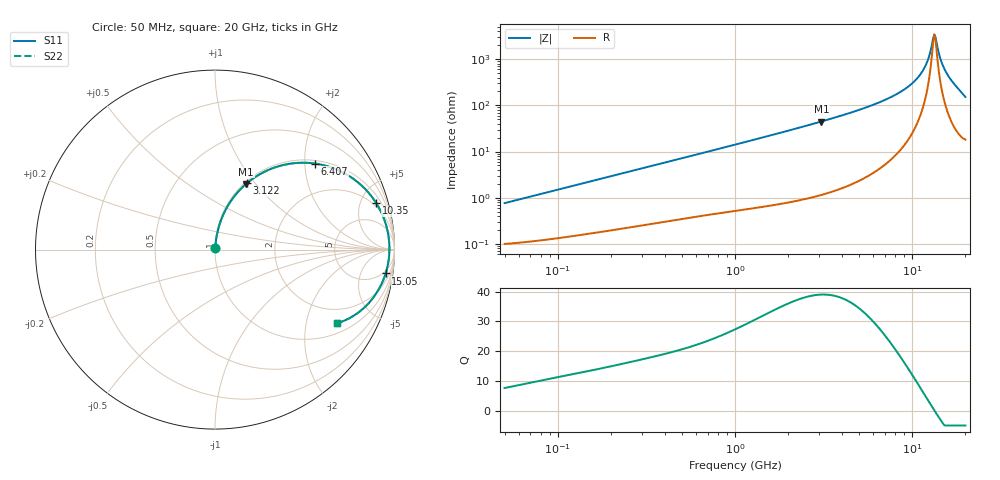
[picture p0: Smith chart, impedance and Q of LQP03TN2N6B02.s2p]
!Murata Part Number: LQP03TN2N6B02
!These Parameters are Measured in Series Mode Connection
!  o--[Z]--o
!Port1  Port2
!  o-------o
!Freq. Start=50[MHz] Stop=20[GHz], 401[Steps]
# Hz S RI R 50
!Freq.(Hz) S11(Real) S11(Imag) S21(Real) S21(Imag) S12(Real) S12(Imag) S22(Real) S22(Imag)
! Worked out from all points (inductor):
!   401 points, 50 MHz to 20 GHz, reference 50 ohm
!   read as one part in series: L = 2.4 nH near 51.52 MHz
!   highest Q = 39 at 3.075 GHz (marker M1), where L = 2.32 nH
!   self-resonance near 13.35 GHz
!   S11 on the Smith chart (normalised r, x): 50 MHz: 1.00, +0.02; 3.122 GHz: 1.02, +0.91; 6.407 GHz: 1.08, +2.26; 10.35 GHz: 1.63, +6.73; 15.05 GHz: 4, -13; 20 GHz: 1.36, -3.02
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5e7  0.00105 0.00755  0.9989 -0.00755  0.9989 -0.00755  0.00105 0.00755
1.364002e8  0.00198 0.0201  0.998 -0.0201  0.998 -0.0201  0.00198 0.0201
3.721004e8  0.0057 0.053  0.9943 -0.053  0.9943 -0.053  0.0057 0.053
1e9  0.0243 0.1367  0.9757 -0.1367  0.9757 -0.1367  0.0243 0.1367
2.728004e9  0.1401 0.3344  0.8599 -0.3344  0.8599 -0.3344  0.1401 0.3344
3.075291e9  0.1732 0.3658  0.8268 -0.3658  0.8268 -0.3658  0.1732 0.3658
3.121702e9  0.1778 0.3697  0.8222 -0.3697  0.8222 -0.3697  0.1778 0.3697
4.472136e9  0.3271 0.4556  0.6729 -0.4556  0.6729 -0.4556  0.3271 0.4556
6.406762e9  0.5583 0.4792  0.4417 -0.4792  0.4417 -0.4792  0.5583 0.4792
7.442007e9  0.672 0.4485  0.328 -0.4485  0.328 -0.4485  0.672 0.4485
8.907419e9  0.8058 0.3667  0.1942 -0.3667  0.1942 -0.3667  0.8058 0.3667
1.034674e10  0.8992 0.2579  0.1008 -0.2579  0.1008 -0.2579  0.8992 0.2579
1.115139e10  0.9342 0.1906  0.0658 -0.1906  0.0658 -0.1906  0.9342 0.1906
1.183995e10  0.9548 0.1315  0.0452 -0.1315  0.0452 -0.1315  0.9548 0.1315
1.238412e10  0.9652 0.0846  0.0348 -0.0846  0.0348 -0.0846  0.9652 0.0846
1.314879e10  0.9717 0.0195  0.0283 -0.0195  0.0283 -0.0195  0.9717 0.0195
1.334722e10  0.9719 0.00283  0.0281 -0.00283  0.0281 -0.00283  0.9719 0.00283
1.375312e10  0.9704 -0.0308  0.0296 0.0308  0.0296 0.0308  0.9704 -0.0308
1.438523e10  0.9636 -0.0818  0.0364 0.0818  0.0364 0.0818  0.9636 -0.0818
1.504638e10  0.9508 -0.1329  0.0492 0.1329  0.0492 0.1329  0.9508 -0.1329
1.696185e10  0.8835 -0.2655  0.1165 0.2655  0.1165 0.2655  0.8835 -0.2655
2e10  0.6788 -0.4106  0.3212 0.4106  0.3212 0.4106  0.6788 -0.4106
